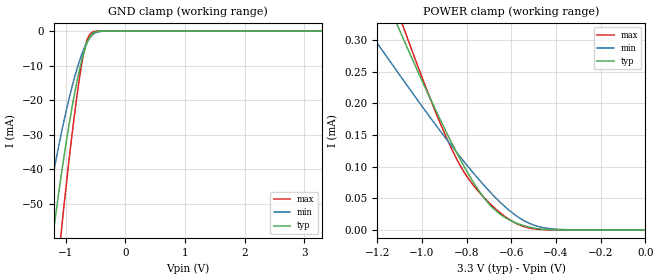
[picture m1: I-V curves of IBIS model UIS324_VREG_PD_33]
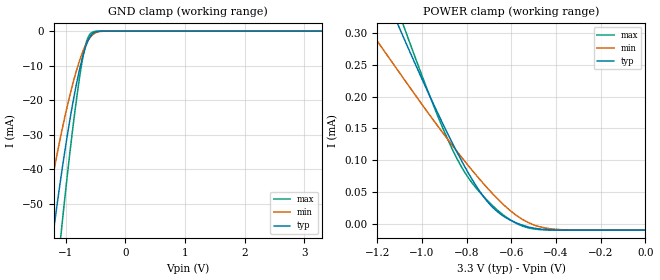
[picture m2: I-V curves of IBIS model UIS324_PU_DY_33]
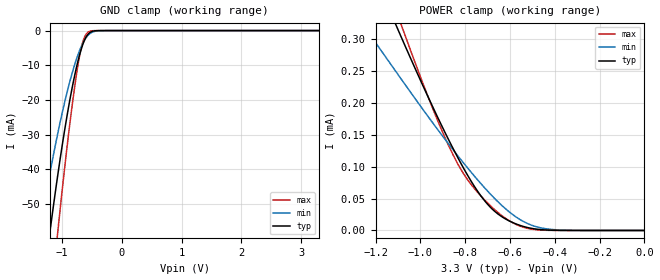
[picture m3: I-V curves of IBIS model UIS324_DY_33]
| TEXAS INSTRUMENTS INCORPORATED
| Connectivity Solutions Department
| IBIS Model of TSB81BA3
| 1394 S800
| This file contains package information for the following:
|  TQFP 80-pin (PFP) package as [Component] TSB81BA3_BETA_PFP
| This device can be powered at the following Vccs:
|  3.3 volt Vcc 1.8 volt Vcc
| This file provides unique models under the [Model Selector] for each Vcc.
| For operation at a specific Vcc, select the appropriate model after each
| [Model Selector] keyword.
[IBIS Ver]   3.2
[Comment char]  |_char
[File Name]   tsb81ba3_rev3p0.ibs
[File Rev]   3.0
[Date]   March 29, 2006
[Source]   Data created from TI-SPICE simulations.
[Notes]   The following is an IBIS list for the TSB81BA3.
[Disclaimer] Property of Texas Instruments Incorporated.  Unauthorized
   reproduction and/or distribution is strictly prohibited.
   This product is protected under copyright law.
   Created  2006, (C) Copyright  2006, Texas Instruments
   Incorporated, All Rights Reserved
   UNLESS THERE IS A SIGNED, WRITTEN AGREEMENT TO THE
   CONTRARY, TEXAS INSTRUMENTS (TI) IS PROVIDING THE IBIS
   MODELS  AND WITHOUT ANY WARRANTY, EXPRESSED OR
   IMPLIED.  TI assumes no liability for:
   1) the accuracy of the IBIS models provided to your
   company;
   2) the proper functioning of these IBIS Models in your
   design or for any resulting applications; or
   3) infringement of patents, copyrights or intellectual
   property rights resulting from your use of these IBIS
   models.
   TI provides IBIS Models as a service to our customers.
   You and your company shall not distribute, sell or give
   these models to anyone else without prior written
   permission from TI.
   TI reserves the right to make changes to our products or
   to discontinue any semiconductor product or service
   without notice, and advises our customers to obtain the
   latest version of relevant information to verify, before
   placing orders, that the information being relied on is
   current.
   Please be aware that your receipt and use of the IBIS
   information provided shall serve as acceptance of these
   terms and conditions.  If you do not accept these terms,
   you should return or destroy the IBIS models and any
   other accompanying information immediately.
| Component TSB81BA3_BETA_PFP 80-pin TQFP
[Component]   TSB81BA3_BETA_PFP
[Manufacturer]   Texas Instruments, Inc.
[Package]
|   typ   min   max
R_pkg   0.1413   0.1318   0.1604
L_pkg   5.561e-09   5.144e-09   6.324e-09
C_pkg   7.967e-13   7.465e-13   8.911e-13
[Pin]   signal_name   model_name   R_pin   L_pin   C_pin
1   PINT   UIS324_OUK831_DY   0.1584   6.267e-09   7.946e-13
2   DS2\LKON   UIS324_OUK831_DY   0.1527   6.022e-09   8.9e-13
3   LREQ   UIS324_PU_DY   0.1478   5.815e-09   8.578e-13
4   DGND   GND   0.1437   5.663e-09   8.22e-13
5   PCLK   UIS324_OUK831_DY   0.1404   5.532e-09   8.02e-13
6   DVDD33HV   POWER   0.1378   5.422e-09   7.874e-13
7   LCLK   UIS324_PU_DY   0.1356   5.325e-09   7.738e-13
8   DVDD18   POWER   0.1342   5.255e-09   7.637e-13
9   CTL0   UIS324_OUK831_DY   0.1334   5.205e-09   7.587e-13
10   CTL1   UIS324_OUK831_DY   0.1332   5.183e-09   7.533e-13
11   D0   UIS324_OUK831_DY   0.1332   5.184e-09   7.532e-13
12   D1   UIS324_OUK831_DY   0.1334   5.207e-09   7.579e-13
13   D2   UIS324_OUK831_DY   0.1342   5.256e-09   7.634e-13
14   DGND   GND   0.1357   5.327e-09   7.738e-13
15   D3   UIS324_OUK831_DY   0.1378   5.423e-09   7.878e-13
16   D4   UIS324_OUK831_DY   0.1405   5.537e-09   8.031e-13
17   D5   UIS324_OUK831_DY   0.1439   5.669e-09   8.216e-13
18   DVDD33HV   POWER   0.1478   5.817e-09   8.431e-13
19   D6   UIS324_OUK831_DY   0.1529   6.029e-09   8.721e-13
20   D7   UIS324_OUK831_DY   0.1586   6.275e-09   7.54e-13
21   AGND   GND   0.1579   6.256e-09   7.932e-13
22   R1   POWER   0.1522   6.009e-09   8.894e-13
23   R0   GND   0.1469   5.793e-09   8.574e-13
24   AVDD33HV   POWER   0.1427   5.637e-09   8.177e-13
25   PLLGND   GND   0.14   5.52e-09   8.011e-13
26   XO   NC   0.1369   5.397e-09   7.894e-13
27   XI   NC   0.1345   5.295e-09   7.747e-13
28   PLLGND   GND   0.133   5.221e-09   7.65e-13
29   PLLVDD18   POWER   0.132   5.168e-09   7.602e-13
30   PLLVDD18   POWER   0.1318   5.144e-09   7.545e-13
31   PLLVDD33HV POWER   0.1318   5.144e-09   7.532e-13
32   DS1   UIS324_DY   0.132   5.167e-09   7.58e-13
33   DS0   UIS324_OUK831_DY   0.1329   5.218e-09   7.643e-13
34   CPS_TD7   UIS324_OUK831_PU   0.1344   5.292e-09   7.733e-13
35   SE   UIS324_PU_DY   0.1365   5.387e-09   7.854e-13
36   SM   UIS324_DY   0.1392   5.499e-09   8.003e-13
37   DVDD18   POWER   0.1425   5.629e-09   8.209e-13
38   DGND   GND   0.1468   5.79e-09   8.567e-13
39   AVDD33HV   POWER   0.1516   5.993e-09   8.88e-13
40   AGND   GND   0.1575   6.246e-09   7.942e-13
41   TPB0_N   DRIVER_SS   0.1591   6.289e-09   7.935e-13
42   TPB0_P   DRIVER_SS   0.1528   6.03e-09   8.868e-13
43   AGND   GND   0.1474   5.809e-09   8.54e-13
44   AVDD33HV   POWER   0.143   5.65e-09   8.161e-13
45   TPA0_N   SSW_IBIS_DRIVERA   0.1395   5.514e-09   7.969e-13
46   TPA0_P   SSW_IBIS_DRIVERA   0.1367   5.399e-09   7.762e-13
47   TPBIAS0   NC   0.1352   5.32e-09   7.605e-13
48   TPB1_N   DRIVER_SS   0.134   5.254e-09   7.56e-13
49   TPB1_P   DRIVER_SS   0.1332   5.205e-09   7.534e-13
50   AGND   GND   0.1332   5.187e-09   7.492e-13
51   AVDD33HV   POWER   0.1335   5.195e-09   7.495e-13
52   TPA1_N   SSW_IBIS_DRIVERA   0.1341   5.229e-09   7.55e-13
53   TPA1_P   SSW_IBIS_DRIVERA   0.1355   5.294e-09   7.574e-13
54   TPBIAS1   NC   0.1369   5.367e-09   7.635e-13
55   TPB2_N   DRIVER_SS   0.1391   5.463e-09   7.814e-13
56   TPB2_P   DRIVER_SS   0.1425   5.593e-09   7.981e-13
57   AVDD33HV   POWER   0.1456   5.719e-09   8.124e-13
58   TPA2_N   SSW_IBIS_DRIVERA   0.1493   5.86e-09   8.507e-13
59   TPA2_P   SSW_IBIS_DRIVERA   0.1549   6.086e-09   8.859e-13
60   TPBIAS2   NC   0.1604   6.324e-09   7.898e-13
61   AGND   GND   0.1578   6.256e-09   7.888e-13
62   AGND   GND   0.1517   6e-09   8.836e-13
63   AVDD33HV   POWER   0.1463   5.782e-09   8.476e-13
64   DGND   GND   0.1428   5.644e-09   8.126e-13
65   DVDD18   POWER   0.1392   5.505e-09   7.941e-13
66   PC0   UIS324_OUK831_DY   0.1366   5.394e-09   7.773e-13
67   PC1   UIS324_OUK831_DY   0.1344   5.299e-09   7.649e-13
68   PC2   UIS324_OUK831_DY   0.1329   5.225e-09   7.556e-13
69   DVDD33HV   POWER   0.132   5.174e-09   7.507e-13
70   DVDD33HV   POWER   0.1318   5.15e-09   7.465e-13
71   DVDD18   POWER   0.1319   5.153e-09   7.465e-13
72   DGND   GND   0.1322   5.18e-09   7.467e-13
73   VREG_PD   UIS324_VREG_PD   0.1329   5.225e-09   7.53e-13
74   BMODE   UIS324_OUK831_DY   0.1346   5.303e-09   7.678e-13
75   RESETZ   UIS324_PU_DY   0.1369   5.403e-09   7.759e-13
76   DGND   GND   0.139   5.501e-09   7.905e-13
77   PD   UIS324_OUK831_DY   0.1425   5.635e-09   8.145e-13
78   TESTM   UIS324_DY   0.1469   5.795e-09   8.514e-13
79   CNA   OUK831_DY   0.1522   6.015e-09   8.834e-13
80   LPS   UIS324_OUK831_DY   0.1578   6.255e-09   7.899e-13
| Model UIS324_VREG_PD
[Model Selector]   UIS324_VREG_PD
UIS324_VREG_PD_33   3.3 volt Vcc
| Model UIS324_PU_DY
[Model Selector]   UIS324_PU_DY
UIS324_PU_DY_33   3.3 volt Vcc
| Model UIS324_DY
[Model Selector]   UIS324_DY
UIS324_DY_33   3.3 volt Vcc
| Model SSW_IBIS_DRIVERA
[Model Selector]   SSW_IBIS_DRIVERA
SSW_IBIS_DRIVERA_33   3.3 volt Vcc
| Model UIS324_OUK831_PU
[Model Selector]   UIS324_OUK831_PU
UIS324_OUK831_PU_33   3.3 volt Vcc
| Model UIS324_OUK831_DY
[Model Selector]   UIS324_OUK831_DY
UIS324_OUK831_DY_33   3.3 volt Vcc
| Model DRIVER_SS
[Model Selector]   DRIVER_SS
DRIVER_SS_33   3.3 volt Vcc
| Model OUK831_DY
[Model Selector]   OUK831_DY
OUK831_DY_33   3.3 volt Vcc
| Models and submodels in the file (8): UIS324_VREG_PD_33 (Input), UIS324_PU_DY_33 (Input), UIS324_DY_33 (Input), SSW_IBIS_DRIVERA_33 (Input), UIS324_OUK831_PU_33 (I/O), UIS324_OUK831_DY_33 (I/O), OUK831_DY_33 (3-state), DRIVER_SS_33 (3-state)
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[Model]   UIS324_VREG_PD_33
Model_type  Input
Vinl=1.05
Vinh=2.34
| variable   typ   min   max
C_comp   1.48pF   0.94pF   3.23pF
[Temperature Range]   40   125   -40
| Ambient temperature   25   110   -40
[Voltage range]   3.3   3   3.6
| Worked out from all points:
|   GND clamp passes 1 mA (typ) near -0.57 V on its own axis
|   POWER clamp passes 1 mA (typ) near -1.93 V on its own axis
[GND Clamp]
| UIS324_VREG_PD_33
|   Voltage   I(typ)   I(min)   I(max)
-3.3V     -411.3mA   -317.3mA   -505.1mA
-1.405V   -85.64mA   -60.8mA    -117.7mA
-1.37V    -80.59mA   -57.17mA   -111.1mA
-1.2V     -57.3mA    -40.59mA   -79.81mA
-1.075V   -41.7mA    -29.67mA   -58.15mA
-890mV    -21.69mA   -15.83mA   -29.33mA
-755mV    -10.14mA   -7.891mA   -11.92mA
-660mV    -4.242mA   -3.807mA   -3.549mA
-615mV    -2.331mA   -2.42mA    -1.48mA
-560mV    -895.4uA   -1.231mA   -374.7uA
-370mV    -7.968uA   -39.26uA   -510.4nA
3.3V      151.5pA    126.7nA    29.06pA
[POWER Clamp]
| UIS324_VREG_PD_33
|   Voltage   I(typ)   I(min)   I(max)
-3.3V     2.151mA    1.417mA    2.424mA
-1.245V   434.1uA    317.5uA    480.7uA
-1.11V    323.6uA    250uA      347uA
-1.085V   303.4uA    237.5uA    322.6uA
-1.065V   287.4uA    227.6uA    303.2uA
-915mV    172uA      154.9uA    166.1uA
-835mV    115.9uA    118.3uA    105.8uA
-740mV    59.33uA    77.65uA    58.13uA
-655mV    26.3uA     45.55uA    28.63uA
-555mV    7.938uA    17.14uA    6.841uA
-455mV    1.149uA    3.601uA    516.5nA
-48.03fV  151.5pA    5.465nA    35.55pA
[Model]   UIS324_PU_DY_33
Model_type  Input
Vinl=1.05
Vinh=2.34
| variable   typ   min   max
C_comp   1.48pF   0.95pF   3.24pF
[Temperature Range]   40   125   -40
| Ambient temperature   25   110   -40
[Voltage range]   3.3   3   3.6
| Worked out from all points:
|   GND clamp passes 1 mA (typ) near -0.56 V on its own axis
|   POWER clamp passes 1 mA (typ) near -1.94 V on its own axis
[GND Clamp]
| UIS324_PU_DY_33
|   Voltage   I(typ)   I(min)   I(max)
-3.3V     -411.3mA   -317.3mA   -505.1mA
-1.405V   -85.64mA   -60.8mA    -117.7mA
-1.37V    -80.6mA    -57.17mA   -111.1mA
-1.2V     -57.3mA    -40.59mA   -79.81mA
-1.075V   -41.7mA    -29.67mA   -58.15mA
-890mV    -21.69mA   -15.84mA   -29.33mA
-755mV    -10.14mA   -7.895mA   -11.93mA
-660mV    -4.248mA   -3.812mA   -3.556mA
-615mV    -2.338mA   -2.425mA   -1.488mA
-560mV    -903.2uA   -1.238mA   -383.5uA
-370mV    -17.92uA   -48.97uA   -10.51uA
3.3V      -10uA      -9.852uA   -10uA
[POWER Clamp]
| UIS324_PU_DY_33
|   Voltage   I(typ)   I(min)   I(max)
-3.3V     2.143mA    1.41mA     2.416mA
-1.24V    421.8uA    307.3uA    467.5uA
-1.11V    315.4uA    242.3uA    338.7uA
-1.085V   295.2uA    229.8uA    314.3uA
-1.065V   279.1uA    219.9uA    294.9uA
-925mV    170.9uA    151.8uA    166uA
-835mV    107.3uA    110.3uA    97.15uA
-735mV    47.93uA    67.4uA     47.24uA
-650mV    15.79uA    35.29uA    17.98uA
-550mV    -2.19uA    6.982uA    -3.449uA
-450mV    -8.878uA   -6.375uA   -9.518uA
-48.03fV  -10uA      -9.995uA   -10uA
[Model]   UIS324_DY_33
Model_type  Input
Vinl=1.05
Vinh=2.34
| variable   typ   min   max
C_comp   1.48pF   0.95pF   3.24pF
[Temperature Range]   40   125   -40
| Ambient temperature   25   110   -40
[Voltage range]   3.3   3   3.6
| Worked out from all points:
|   GND clamp passes 1 mA (typ) near -0.57 V on its own axis
|   POWER clamp passes 1 mA (typ) near -1.93 V on its own axis
[GND Clamp]
| UIS324_DY_33
|   Voltage   I(typ)   I(min)   I(max)
-3.3V     -411.3mA   -317.3mA   -505.1mA
-1.405V   -85.64mA   -60.8mA    -117.7mA
-1.37V    -80.59mA   -57.17mA   -111.1mA
-1.2V     -57.3mA    -40.59mA   -79.81mA
-1.075V   -41.7mA    -29.67mA   -58.15mA
-890mV    -21.69mA   -15.83mA   -29.33mA
-755mV    -10.14mA   -7.891mA   -11.92mA
-660mV    -4.242mA   -3.807mA   -3.549mA
-615mV    -2.331mA   -2.42mA    -1.48mA
-560mV    -895.4uA   -1.231mA   -374.7uA
-370mV    -7.968uA   -39.26uA   -510.4nA
3.3V      151.5pA    126.7nA    29.06pA
[POWER Clamp]
| UIS324_DY_33
|   Voltage   I(typ)   I(min)   I(max)
-3.3V     2.151mA    1.417mA    2.424mA
-1.245V   434.1uA    317.5uA    480.7uA
-1.11V    323.6uA    250uA      347uA
-1.085V   303.4uA    237.5uA    322.6uA
-1.065V   287.4uA    227.6uA    303.2uA
-915mV    172uA      154.9uA    166.1uA
-835mV    115.9uA    118.3uA    105.8uA
-740mV    59.33uA    77.65uA    58.13uA
-655mV    26.3uA     45.55uA    28.63uA
-555mV    7.938uA    17.14uA    6.841uA
-455mV    1.149uA    3.601uA    516.5nA
-48.03fV  151.5pA    5.465nA    35.55pA
